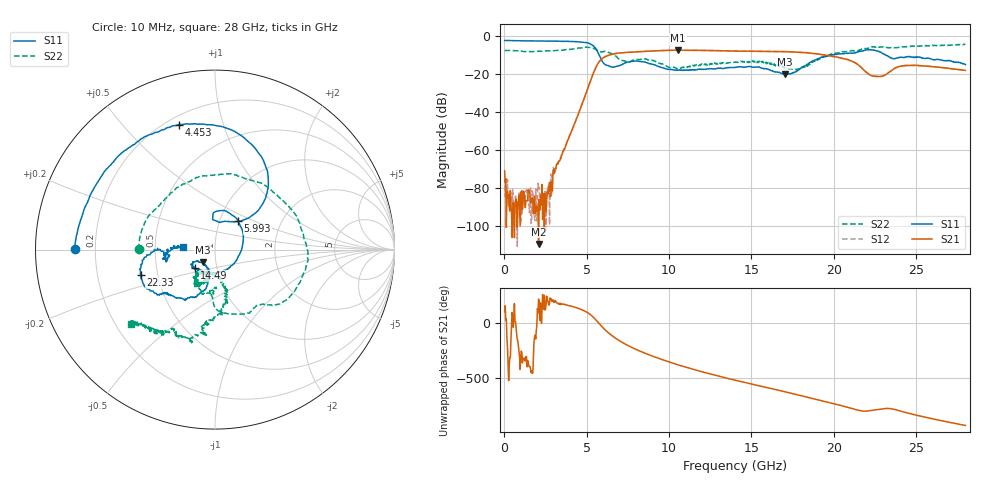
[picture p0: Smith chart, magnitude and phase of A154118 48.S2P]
!  2-Port S-parameters saved by WinCal
! VAR MeasName=S-Parameters (CALIBRATED_DATA) read from VNA (N5230A)
! VAR MeasDate=2015-9-10 14:38:12
! VAR NAME=A154118 48
! VAR FILENAME=A154118 48.S2P
! VAR DATE=2015-9-10 14:38:12
! VAR PHYS_PORTS=1,2
# Hz S DB R 50
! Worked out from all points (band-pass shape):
!   801 points, 10 MHz to 28 GHz, reference 50 ohm
!   highest |S21| = -7.29 dB at 10.54 GHz (marker M1); lowest = -109.8 dB at 2.074 GHz (marker M2)
!   |S21| within 3 dB of the highest: 6.228 GHz to 19.76 GHz (13.53 GHz wide, 104 % of centre)
!   lowest |S11| = -20.1 dB at 17.01 GHz (marker M3), VSWR 1.22, Z = 43.2 - j6.2 ohm
!   |S11| at or under -10 dB: 5.763 GHz to 19.74 GHz (13.98 GHz wide, 110 % of centre); 23.21 GHz to end of sweep
!   |S22| runs from -17.6 to -4.1 dB; largest |S21 - S12| = 0.0078
!   S11 on the Smith chart (normalised r, x): 10 MHz: 0.12, +0.00; 4.453 GHz: 0.25, +0.72; 5.993 GHz: 1.22, +0.40; 14.49 GHz: 0.78, -0.16; 22.33 GHz: 0.40, -0.14; 28 GHz: 0.70, +0.02
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1e7  -2.15 179.7  -71.09 99.8  -78.56 -77.6  -7.49 179.8
2.549125e8  -2.18 176.2  -83.70 -163.9  -85.81 51.1  -7.44 172.1
2.074262e9  -2.43 152.5  -109.77 -145.8  -81.33 130.9  -7.87 120.5
2.774012e9  -2.49 142.1  -81.60 -136.0  -80.28 -164.3  -7.67 97.3
4.453412e9  -2.79 106.1  -41.82 131.5  -41.74 131.7  -6.21 23.2
4.698325e9  -3.03 98.0  -36.21 118.3  -36.16 118.1  -6.03 9.7
5.46805e9  -5.57 56.3  -18.06 40.2  -18.08 40.3  -6.48 -39.7
5.992862e9  -13.82 50.8  -11.37 -46.4  -11.38 -46.5  -8.00 -58.5
6.517675e9  -16.13 78.9  -9.49 -114.7  -9.49 -115.1  -9.10 -84.2
7.2874e9  -14.23 93.4  -8.55 171.0  -8.57 170.9  -12.98 -92.5
8.26705e9  -13.32 64.9  -8.06 101.1  -8.05 100.9  -12.12 -100.5
9.351662e9  -15.90 13.4  -7.58 38.8  -7.55 38.7  -14.16 -123.3
1.054124e10  -17.76 -53.1  -7.29 -20.6  -7.28 -20.9  -17.32 -112.5
1.215066e10  -17.35 -112.8  -7.44 -89.3  -7.40 -89.9  -14.66 -106.9
1.4005e10  -16.46 -133.4  -7.75 -159.1  -7.73 -159.6  -13.67 -113.2
1.449482e10  -16.31 -138.3  -7.80 -176.1  -7.82 -176.6  -13.49 -112.6
1.701392e10  -20.11 -133.9  -8.09 96.8  -8.10 96.4  -16.23 -119.5
1.869332e10  -13.09 -102.9  -8.97 35.6  -8.97 35.1  -13.24 -75.4
2.079258e10  -9.04 -134.9  -12.14 -42.7  -12.07 -43.3  -8.04 -93.6
2.233202e10  -7.18 -161.3  -20.85 -72.4  -20.93 -73.1  -5.57 -103.9
2.334666e10  -10.79 -178.1  -19.08 -55.2  -19.08 -55.8  -6.05 -117.0
2.8e10  -14.89 175.3  -17.97 151.2  -18.01 150.7  -4.09 -138.6
